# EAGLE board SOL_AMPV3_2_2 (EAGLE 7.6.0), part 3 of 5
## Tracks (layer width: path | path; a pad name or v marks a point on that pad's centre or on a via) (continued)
D13:N$7  (via drill 0.4) (continued)
  BOTTOM 0.254: D13:C35.2 44.85,129.65 44.83,129.67 44.83,129.91 | 44.83,129.91 D13:R39.1 | 44.83,129.91 47.55,129.91 v47.69,130.05
D13:N$10
  Top 0.406: D13:R41.1 30.97,127.93 D13:C41.1
D13:R31
  Top 0.406: D13:R31.1 30.97,135.03 D13:C31.1
D13:VB+
  Top 0.406: D13:R37.2 27.05,133.22 27.37,132.91 27.37,132.59 | 27.37,132.59 27.37,131.97 D13:R36.1 | D13:C36.1 27.37,132.59
D13:VB-  (via drill 0.4)
  Top 0.406: D13:C46.1 28.74,130.68 D13:R46.2 27.37,130.67 27.37,129.73 27.05,129.41 D13:R47.1 26.84,129.09 v25.46,129.41
  BOTTOM 0.406: D13:R50.2 25.48,129.43 v25.46,129.41
D13:VCOM  (via drill 0.4)
  Top 0.254: D13:U1.2 41.33,130.03 41.34,130.05 41.34,130.37 41.02,130.68 v39.43,131
  BOTTOM 0.254: v39.43,131 D13:C7.1 38.19,129.11 D13:R1.2
D14:AMP+
  Top 0.254: 89.58,113.84 86.42,113.86 86.12,114.16 D14:C43.2 85.38,114.16 D14:R43.2 | 89.58,113.84 89.6,114.49 89.6,115.3 D14:U1.4 | 89.58,113.84 89.6,113.86 D14:C44.1 D14:R44.1 D14:R61.2
D14:AMP-
  Top 0.254: D14:R33.2 85.35,120.22 D14:C33.2 86.44,120.22 87.06,120.84 89.61,120.84 | 89.61,120.84 D14:U1.5 | 89.61,120.84 91.49,120.84 D14:R34.1 D14:C34.1 D14:R51.2
D14:FB+
  Top 0.254: D14:R32.1 D14:R33.1 81.66,120.84 D14:C32.2 D14:R31.2
D14:FB-
  Top 0.254: D14:R43.1 83.03,115.44 | 83.03,115.44 D14:R42.1 | D14:R41.2 D14:C42.2 81.66,115.44 83.03,115.44
D14:N$1  (via drill 0.4)
  Top 0.254: D14:R51.1 93.61,117.98 | 93.61,117.98 D14:R45.1 | v94.36,117.98 93.61,117.98
  BOTTOM 0.254: v94.36,117.98 94.09,118.25 D14:R49.1 93.11,118.27 D14:C45.2
D14:N$4
  Top 0.254: D14:U1.1 85.96,115.32 D14:C43.1 85.77,115.14 84.84,116.08 D14:R42.2
D14:N$5
  Top 0.254: D14:U1.8 87.5,119.38 87.38,119.25 87.06,119.25 86.74,118.94 86.12,118.94 D14:C33.1 85.04,118.92 D14:R32.2
D14:N$7  (via drill 0.4)
  Top 0.254: D14:R61.1 v94.68,116.08 95.31,116.71 95.31,118.62 D14:R35.2
  BOTTOM 0.254: v94.68,116.08 93.41,114.81 D14:C35.2 91.82,114.82 91.82,116.08 91.58,116.32 D14:R39.1
D14:N$10
  Top 0.406: D14:R41.1 77.96,113.96 D14:C41.1
D14:R31
  Top 0.406: D14:R31.1 77.96,121.06 D14:C31.1
D14:VB+
  Top 0.406: D14:R37.2 74.04,119.25 74.36,118.94 74.36,118.62 | 74.36,118.62 74.36,118 D14:R36.1 | D14:C36.1 74.36,118.62
D14:VB-  (via drill 0.4)
  Top 0.406: D14:C46.1 75.73,116.71 D14:R46.2 74.36,116.7 74.36,115.76 74.04,115.44 D14:R47.1 73.83,115.13 v72.45,115.44
  BOTTOM 0.406: D14:R50.2 72.47,115.46 v72.45,115.44
D14:VCOM  (via drill 0.4)
  Top 0.254: D14:U1.2 88.32,116.06 88.33,116.08 88.33,116.39 88.01,116.71 v86.42,117.03
  BOTTOM 0.254: v86.42,117.03 D14:C7.1 85.18,115.14 D14:R1.2
D15:AMP+
  Top 0.254: 42.59,115.11 39.43,115.13 39.13,115.43 D15:C43.2 38.39,115.43 D15:R43.2 | 42.59,115.11 42.61,115.76 42.61,116.57 D15:U1.4 | 42.59,115.11 42.61,115.13 D15:C44.1 D15:R44.1 D15:R61.2
D15:AMP-
  Top 0.254: D15:R33.2 38.36,121.49 D15:C33.2 39.45,121.49 40.07,122.11 42.62,122.11 | 42.62,122.11 D15:U1.5 | 42.62,122.11 44.5,122.11 D15:R34.1 D15:C34.1 D15:R51.2
D15:FB+
  Top 0.254: D15:R32.1 D15:R33.1 34.67,122.11 D15:C32.2 D15:R31.2
D15:FB-
  Top 0.254: D15:R43.1 36.04,116.71 | 36.04,116.71 D15:R42.1 | D15:R41.2 D15:C42.2 34.67,116.71 36.04,116.71
D15:N$1  (via drill 0.4)
  Top 0.254: D15:R51.1 46.62,119.25 | 46.62,119.25 D15:R45.1 | v47.37,119.25 46.62,119.25
  BOTTOM 0.254: D15:C45.2 46.1,121.14 D15:R49.1 47.1,119.52 v47.37,119.25
D15:N$4
  Top 0.254: D15:U1.1 38.97,116.59 D15:C43.1 38.78,116.41 37.85,117.35 D15:R42.2
D15:N$5
  Top 0.254: D15:U1.8 40.51,120.65 40.39,120.52 40.07,120.52 39.75,120.21 39.13,120.21 D15:C33.1 38.05,120.19 D15:R32.2
D15:N$7  (via drill 0.4)
  Top 0.254: D15:R61.1 v47.69,117.35 48.32,117.98 48.32,119.89 D15:R35.2
  BOTTOM 0.254: D15:R39.1 44.59,117.71 44.96,117.35 44.96,116.19 D15:C35.2 46.42,116.08 v47.69,117.35
D15:N$10
  Top 0.406: D15:R41.1 30.97,115.23 D15:C41.1
D15:R31
  Top 0.406: D15:R31.1 30.97,122.33 D15:C31.1
D15:VB+
  Top 0.406: D15:R37.2 27.05,120.52 27.37,120.21 27.37,119.89 | 27.37,119.89 27.37,119.27 D15:R36.1 | D15:C36.1 27.37,119.89
D15:VB-  (via drill 0.4)
  Top 0.406: D15:C46.1 28.74,117.98 D15:R46.2 27.37,117.97 27.37,117.03 27.05,116.71 D15:R47.1 26.84,116.39 v25.46,116.71
  BOTTOM 0.406: D15:R50.2 25.48,116.73 v25.46,116.71
D15:VCOM  (via drill 0.4)
  Top 0.254: D15:U1.2 41.33,117.33 41.34,117.35 41.34,117.67 41.02,117.98 v39.43,118.3
  BOTTOM 0.254: v39.43,118.3 D15:C7.1 38.19,116.41 D15:R1.2
D16:AMP+
  Top 0.254: 42.59,98.6 39.43,98.61 39.13,98.92 D16:C43.2 38.39,98.92 D16:R43.2 | 42.59,98.6 42.61,99.25 42.61,100.06 D16:U1.4 | 42.59,98.6 42.61,98.61 D16:C44.1 D16:R44.1 D16:R61.2
D16:AMP-
  Top 0.254: D16:R33.2 38.36,104.98 D16:C33.2 39.45,104.98 40.07,105.6 42.62,105.6 | 42.62,105.6 D16:U1.5 | 42.62,105.6 44.5,105.6 D16:R34.1 D16:C34.1 D16:R51.2
D16:FB+
  Top 0.254: D16:R32.1 D16:R33.1 34.67,105.6 D16:C32.2 D16:R31.2
D16:FB-
  Top 0.254: D16:R43.1 36.04,100.2 | 36.04,100.2 D16:R42.1 | D16:R41.2 D16:C42.2 34.67,100.2 36.04,100.2
D16:N$1  (via drill 0.4)
  Top 0.254: D16:R51.1 46.62,102.74 | 46.62,102.74 D16:R45.1 | v47.37,102.74 46.62,102.74
  BOTTOM 0.254: v47.37,102.74 47.1,103.01 D16:R49.1 46.12,103.03 D16:C45.2
D16:N$4
  Top 0.254: D16:U1.1 38.97,100.08 D16:C43.1 38.78,99.9 37.85,100.84 D16:R42.2
D16:N$5
  Top 0.254: D16:U1.8 40.51,104.14 40.39,104.01 40.07,104.01 39.75,103.69 39.13,103.69 D16:C33.1 38.05,103.68 D16:R32.2
D16:N$7  (via drill 0.4)
  Top 0.254: D16:R61.1 v47.69,100.84 48.32,101.47 48.32,103.38 D16:R35.2
  BOTTOM 0.254: D16:R39.1 44.59,101.08 44.83,100.84 | 44.83,100.84 44.83,99.58 D16:C35.2 | 44.83,100.84 v47.69,100.84
D16:N$10
  Top 0.406: D16:R41.1 30.97,98.72 D16:C41.1
D16:R31
  Top 0.406: D16:R31.1 30.97,105.82 D16:C31.1
D16:VB+
  Top 0.406: D16:R37.2 27.05,104.01 27.37,103.69 27.37,103.38 | 27.37,103.38 27.37,102.76 D16:R36.1 | D16:C36.1 27.37,103.38
D16:VB-  (via drill 0.4)
  Top 0.406: D16:C46.1 28.74,101.47 D16:R46.2 27.37,101.46 27.37,100.52 27.05,100.2 D16:R47.1 26.84,99.89 v25.46,100.2
  BOTTOM 0.406: D16:R50.2 25.48,100.22 v25.46,100.2
D16:VCOM  (via drill 0.4)
  Top 0.254: D16:U1.2 41.33,100.83 41.34,100.84 41.34,101.16 41.02,101.47 v39.43,101.79
  BOTTOM 0.254: v39.43,101.79 D16:C7.1 38.19,99.9 D16:R1.2
D17:AMP+
  Top 0.254: 78.79,95.68 75.63,95.69 75.33,96 D17:C43.2 74.59,96 D17:R43.2 | 78.79,95.68 78.8,96.33 78.8,97.14 D17:U1.4 | 78.79,95.68 78.8,95.69 D17:C44.1 D17:R44.1 D17:R61.2
D17:AMP-
  Top 0.254: D17:R33.2 74.56,102.06 D17:C33.2 75.64,102.06 76.26,102.68 78.82,102.68 | 78.82,102.68 D17:U1.5 | 78.82,102.68 80.69,102.68 D17:R34.1 D17:C34.1 D17:R51.2
D17:FB+
  Top 0.254: D17:R32.1 D17:R33.1 70.87,102.68 D17:C32.2 D17:R31.2
D17:FB-
  Top 0.254: D17:R43.1 72.24,97.28 | 72.24,97.28 D17:R42.1 | D17:R41.2 D17:C42.2 70.87,97.28 72.24,97.28
D17:N$1  (via drill 0.4)
  Top 0.254: D17:R51.1 82.82,99.82 | 82.82,99.82 D17:R45.1 | v83.57,99.82 82.82,99.82
  BOTTOM 0.254: v83.57,99.82 83.3,100.09 D17:R49.1 82.31,100.11 D17:C45.2
D17:N$4
  Top 0.254: D17:U1.1 75.17,97.16 D17:C43.1 74.98,96.98 74.04,97.92 D17:R42.2
D17:N$5
  Top 0.254: D17:U1.8 76.71,101.22 76.58,101.09 76.26,101.09 75.95,100.78 75.33,100.78 D17:C33.1 74.24,100.76 D17:R32.2
D17:N$7  (via drill 0.4)
  Top 0.254: D17:R61.1 v83.88,97.92 84.52,98.55 84.52,100.46 D17:R35.2
  BOTTOM 0.305: D17:C35.2 81.03,97.66 81.03,97.92 | D17:R39.1 81.03,97.92 | 81.03,97.92 v83.88,97.92
D17:N$10
  Top 0.406: D17:R41.1 67.17,95.8 D17:C41.1
D17:R31
  Top 0.406: D17:R31.1 67.17,102.89 D17:C31.1
D17:VB+
  Top 0.406: D17:R37.2 63.25,101.09 63.56,100.78 63.56,100.46 | 63.56,100.46 63.56,99.84 D17:R36.1 | D17:C36.1 63.56,100.46
D17:VB-  (via drill 0.4)
  Top 0.406: D17:C46.1 64.94,98.55 D17:R46.2 63.56,98.54 63.56,97.6 63.25,97.28 D17:R47.1 63.03,96.97 v61.66,97.28
  BOTTOM 0.406: D17:R50.2 61.67,97.3 v61.66,97.28
D17:VCOM  (via drill 0.4)
  Top 0.254: D17:U1.2 77.52,97.9 77.53,97.92 77.53,98.23 77.22,98.55 v75.63,98.87
  BOTTOM 0.254: v75.63,98.87 D17:C7.1 74.39,96.98 D17:R1.2
D18:AMP+
  Top 0.254: 42.59,87.42 39.43,87.44 39.13,87.74 D18:C43.2 38.39,87.74 D18:R43.2 | 42.59,87.42 42.61,88.08 42.61,88.89 D18:U1.4 | 42.59,87.42 42.61,87.44 D18:C44.1 D18:R44.1 D18:R61.2
D18:AMP-
  Top 0.254: D18:R33.2 38.36,93.81 D18:C33.2 39.45,93.81 40.07,94.42 42.62,94.42 | 42.62,94.42 D18:U1.5 | 42.62,94.42 44.5,94.42 D18:R34.1 D18:C34.1 D18:R51.2
D18:FB+
  Top 0.254: D18:R32.1 D18:R33.1 34.67,94.42 D18:C32.2 D18:R31.2
D18:FB-
  Top 0.254: D18:R43.1 36.04,89.03 | 36.04,89.03 D18:R42.1 | D18:R41.2 D18:C42.2 34.67,89.03 36.04,89.03
D18:N$1  (via drill 0.4)
  Top 0.254: D18:R51.1 46.62,91.57 | 46.62,91.57 D18:R45.1 | v47.37,91.57 46.62,91.57
  BOTTOM 0.254: D18:C45.2 46.12,91.85 D18:R49.1
  BOTTOM 0.305: D18:R49.1 v47.37,91.57
D18:N$4
  Top 0.254: D18:U1.1 38.97,88.9 D18:C43.1 38.78,88.72 37.85,89.66 D18:R42.2
D18:N$5
  Top 0.254: D18:U1.8 40.51,92.96 40.39,92.84 40.07,92.84 39.75,92.52 39.13,92.52 D18:C33.1 38.05,92.5 D18:R32.2
D18:N$7  (via drill 0.4)
  Top 0.254: D18:R61.1 v47.69,89.66 48.32,90.3 48.32,92.2 D18:R35.2
  BOTTOM 0.254: D18:R39.1 44.96,89.41 | 44.96,89.41 44.96,88.5 D18:C35.2 | 44.96,89.41 47.43,89.41 v47.69,89.66
D18:N$10
  Top 0.406: D18:R41.1 30.97,87.54 D18:C41.1
D18:R31
  Top 0.406: D18:R31.1 30.97,94.64 D18:C31.1
D18:VB+
  Top 0.406: D18:R37.2 27.05,92.84 27.37,92.52 27.37,92.2 | 27.37,92.2 27.37,91.58 D18:R36.1 | D18:C36.1 27.37,92.2
D18:VB-  (via drill 0.4)
  Top 0.406: D18:C46.1 28.74,90.3 D18:R46.2 27.37,90.28 27.37,89.34 27.05,89.03 D18:R47.1 26.84,88.71 v25.46,89.03
  BOTTOM 0.406: D18:R50.2 25.48,89.04 v25.46,89.03
D18:VCOM  (via drill 0.4)
  Top 0.254: D18:U1.2 41.33,89.65 41.34,89.66 41.34,89.98 41.02,90.3 v39.43,90.61
  BOTTOM 0.254: v39.43,90.61 D18:C7.1 38.19,88.72 D18:R1.2
D19:AMP+
  Top 0.254: 78.79,84.25 75.63,84.26 75.33,84.57 D19:C43.2 74.59,84.57 D19:R43.2 | 78.79,84.25 78.8,84.9 78.8,85.71 D19:U1.4 | 78.79,84.25 78.8,84.26 D19:C44.1 D19:R44.1 D19:R61.2
D19:AMP-
  Top 0.254: D19:R33.2 74.56,90.63 D19:C33.2 75.64,90.63 76.26,91.25 78.82,91.25 | 78.82,91.25 D19:U1.5 | 78.82,91.25 80.69,91.25 D19:R34.1 D19:C34.1 D19:R51.2
D19:FB+
  Top 0.254: D19:R32.1 D19:R33.1 70.87,91.25 D19:C32.2 D19:R31.2
D19:FB-
  Top 0.254: D19:R43.1 72.24,85.85 | 72.24,85.85 D19:R42.1 | D19:R41.2 D19:C42.2 70.87,85.85 72.24,85.85
D19:N$1  (via drill 0.4)
  Top 0.254: D19:R51.1 82.82,88.39 | 82.82,88.39 D19:R45.1 | v83.57,88.39 82.82,88.39
  BOTTOM 0.254: v83.57,88.39 83.3,88.66 D19:R49.1 82.31,88.68 D19:C45.2
D19:N$4
  Top 0.254: D19:U1.1 75.17,85.72 D19:C43.1 74.98,85.55 74.04,86.49 D19:R42.2
D19:N$5
  Top 0.254: D19:U1.8 76.71,89.79 76.58,89.66 76.26,89.66 75.95,89.34 75.33,89.34 D19:C33.1 74.24,89.33 D19:R32.2
D19:N$7  (via drill 0.4)
  Top 0.254: D19:R61.1 v83.88,86.49 84.52,87.12 84.52,89.03 D19:R35.2
  BOTTOM 0.254: D19:C35.2 80.9,85.47 80.9,86.47 D19:R39.1 81.39,86.73 81.41,86.74 81.66,86.49 v83.88,86.49
D19:N$10
  Top 0.406: D19:R41.1 67.17,84.37 D19:C41.1
D19:R31
  Top 0.406: D19:R31.1 67.17,91.47 D19:C31.1
D19:VB+
  Top 0.406: D19:R37.2 63.25,89.66 63.56,89.34 63.56,89.03 | 63.56,89.03 63.56,88.41 D19:R36.1 | D19:C36.1 63.56,89.03
D19:VB-  (via drill 0.4)
  Top 0.406: D19:C46.1 64.94,87.12 D19:R46.2 63.56,87.11 63.56,86.17 63.25,85.85 D19:R47.1 63.03,85.53 v61.66,85.85
  BOTTOM 0.406: D19:R50.2 61.67,85.87 v61.66,85.85
D19:VCOM  (via drill 0.4)
  Top 0.254: D19:U1.2 77.52,86.47 77.53,86.49 77.53,86.81 77.22,87.12 v75.63,87.44
  BOTTOM 0.254: v75.63,87.44 D19:C7.1 74.39,85.55 D19:R1.2
D20:AMP+
  Top 0.254: 43.86,71.93 40.7,71.94 40.4,72.25 D20:C43.2 39.66,72.25 D20:R43.2 | 43.86,71.93 43.88,72.58 43.88,73.39 D20:U1.4 | 43.86,71.93 43.88,71.94 D20:C44.1 D20:R44.1 D20:R61.2
D20:AMP-
  Top 0.254: D20:R33.2 39.63,78.31 D20:C33.2 40.72,78.31 41.34,78.93 43.89,78.93 | 43.89,78.93 D20:U1.5 | 43.89,78.93 45.77,78.93 D20:R34.1 D20:C34.1 D20:R51.2
D20:FB+
  Top 0.254: D20:R32.1 D20:R33.1 35.94,78.93 D20:C32.2 D20:R31.2
D20:FB-
  Top 0.254: D20:R43.1 37.31,73.53 | 37.31,73.53 D20:R42.1 | D20:R41.2 D20:C42.2 35.94,73.53 37.31,73.53
D20:N$1  (via drill 0.4)
  Top 0.254: D20:R51.1 47.89,76.07 | 47.89,76.07 D20:R45.1 | v48.64,76.07 47.89,76.07
  BOTTOM 0.254: v48.64,76.07 48.37,76.34 D20:R49.1 47.39,76.36 D20:C45.2
D20:N$4
  Top 0.254: D20:U1.1 40.24,73.41 D20:C43.1 40.05,73.23 39.12,74.17 D20:R42.2
D20:N$5
  Top 0.254: D20:U1.8 41.78,77.47 41.66,77.34 41.34,77.34 41.02,77.03 40.4,77.03 D20:C33.1 39.32,77.01 D20:R32.2
D20:N$7  (via drill 0.4)
  Top 0.254: D20:R61.1 v48.96,74.17 49.59,74.8 49.59,76.71 D20:R35.2
  BOTTOM 0.254: 45.97,74.17 45.97,73.04 D20:C35.2 | D20:R39.1 45.73,74.41 45.97,74.17 | 45.97,74.17 v48.96,74.17
D20:N$10
  Top 0.406: D20:R41.1 32.24,72.05 D20:C41.1
D20:R31
  Top 0.406: D20:R31.1 32.24,79.14 D20:C31.1
D20:VB+
  Top 0.406: D20:R37.2 28.32,77.34 28.64,77.03 28.64,76.71 | 28.64,76.71 28.64,76.09 D20:R36.1 | D20:C36.1 28.64,76.71
D20:VB-  (via drill 0.4)
  Top 0.406: D20:C46.1 30.01,74.8 D20:R46.2 28.64,74.79 28.64,73.85 28.32,73.53 D20:R47.1 28.11,73.22 v26.73,73.53
  BOTTOM 0.406: D20:R50.2 26.75,73.55 v26.73,73.53
D20:VCOM  (via drill 0.4)
  Top 0.254: D20:U1.2 42.6,74.16 42.61,74.17 42.61,74.49 42.29,74.8 v40.7,75.12
  BOTTOM 0.254: v40.7,75.12 D20:C7.1 39.46,73.23 D20:R1.2
D21:AMP+
  Top 0.254: 85.77,69.39 82.61,69.41 82.31,69.71 D21:C43.2 81.57,69.71 D21:R43.2 | 85.77,69.39 85.79,70.04 85.79,70.85 D21:U1.4 | 85.77,69.39 85.79,69.41 D21:C44.1 D21:R44.1 D21:R61.2
D21:AMP-
  Top 0.254: D21:R33.2 81.54,75.77 D21:C33.2 82.63,75.77 83.25,76.39 85.8,76.39 | 85.8,76.39 D21:U1.5 | 85.8,76.39 87.68,76.39 D21:R34.1 D21:C34.1 D21:R51.2
D21:FB+
  Top 0.254: D21:R32.1 D21:R33.1 77.85,76.39 D21:C32.2 D21:R31.2
D21:FB-
  Top 0.254: D21:R43.1 79.22,70.99 | 79.22,70.99 D21:R42.1 | D21:R41.2 D21:C42.2 77.85,70.99 79.22,70.99
D21:N$1  (via drill 0.4)
  Top 0.254: D21:R51.1 89.8,73.53 | 89.8,73.53 D21:R45.1 | v90.55,73.53 89.8,73.53
  BOTTOM 0.254: v90.55,73.53 90.28,73.8 D21:R49.1 89.3,73.83 D21:C45.2
D21:N$4
  Top 0.254: D21:U1.1 82.15,70.87 D21:C43.1 81.96,70.69 81.03,71.63 D21:R42.2
D21:N$5
  Top 0.254: D21:U1.8 83.69,74.93 83.57,74.8 83.25,74.8 82.93,74.49 82.31,74.49 D21:C33.1 81.23,74.47 D21:R32.2
D21:N$7  (via drill 0.4)
  Top 0.254: D21:R61.1 v90.87,71.63 91.5,72.26 91.5,74.17 D21:R35.2
  BOTTOM 0.254: D21:C35.2 87.88,70.5 87.88,71.63 87.63,71.63 D21:R39.1 87.87,71.63 v90.87,71.63
D21:N$10
  Top 0.406: D21:R41.1 74.15,69.51 D21:C41.1
D21:R31
  Top 0.406: D21:R31.1 74.15,76.61 D21:C31.1
D21:VB+
  Top 0.406: D21:R37.2 70.23,74.8 70.55,74.49 70.55,74.17 | 70.55,74.17 70.55,73.55 D21:R36.1 | D21:C36.1 70.55,74.17
D21:VB-  (via drill 0.4)
  Top 0.406: D21:C46.1 71.92,72.26 D21:R46.2 70.55,72.25 70.55,71.31 70.23,70.99 D21:R47.1 70.02,70.67 v68.64,70.99
  BOTTOM 0.406: D21:R50.2 68.66,71.01 v68.64,70.99
D21:VCOM  (via drill 0.4)
  Top 0.254: D21:U1.2 84.51,71.61 84.52,71.63 84.52,71.94 84.2,72.26 v82.61,72.58
  BOTTOM 0.254: v82.61,72.58 D21:C7.1 81.37,70.69 D21:R1.2
D22:AMP+
  Top 0.254: 42.59,60.5 39.43,60.52 39.13,60.82 D22:C43.2 38.39,60.82 D22:R43.2 | 42.59,60.5 42.61,61.15 42.61,61.96 D22:U1.4 | 42.59,60.5 42.61,60.52 D22:C44.1 D22:R44.1 D22:R61.2
D22:AMP-
  Top 0.254: D22:R33.2 38.36,66.88 D22:C33.2 39.45,66.88 40.07,67.5 42.62,67.5 | 42.62,67.5 D22:U1.5 | 42.62,67.5 44.5,67.5 D22:R34.1 D22:C34.1 D22:R51.2
D22:FB+
  Top 0.254: D22:R32.1 D22:R33.1 34.67,67.5 D22:C32.2 D22:R31.2
D22:FB-
  Top 0.254: D22:R43.1 36.04,62.1 | 36.04,62.1 D22:R42.1 | D22:R41.2 D22:C42.2 34.67,62.1 36.04,62.1
D22:N$1  (via drill 0.4)
  Top 0.254: D22:R51.1 46.62,64.64 | 46.62,64.64 D22:R45.1 | v47.37,64.64 46.62,64.64
  BOTTOM 0.254: D22:C45.2 46.1,66.53 D22:R49.1 47.1,64.91 v47.37,64.64
D22:N$4
  Top 0.254: D22:U1.1 38.97,61.98 D22:C43.1 38.78,61.8 37.85,62.74 D22:R42.2
D22:N$5
  Top 0.254: D22:U1.8 40.51,66.04 40.39,65.91 40.07,65.91 39.75,65.6 39.13,65.6 D22:C33.1 38.05,65.58 D22:R32.2
D22:N$7  (via drill 0.4)
  Top 0.254: D22:R61.1 v47.69,62.74 48.32,63.37 48.32,65.28 D22:R35.2
  BOTTOM 0.254: D22:R39.1 44.45,62.99 44.83,62.61 | 44.83,62.61 44.83,61.48 D22:C35.2 | 44.83,62.61 45.99,62.61 D22:R61.1 v47.69,62.74
D22:N$10
  Top 0.406: D22:R41.1 30.97,60.62 D22:C41.1
D22:R31
  Top 0.406: D22:R31.1 30.97,67.72 D22:C31.1
D22:VB+
  Top 0.406: D22:R37.2 27.05,65.91 27.37,65.6 27.37,65.28 | 27.37,65.28 27.37,64.66 D22:R36.1 | D22:C36.1 27.37,65.28
D22:VB-  (via drill 0.4)
  Top 0.406: D22:C46.1 28.74,63.37 D22:R46.2 27.37,63.36 27.37,62.42 27.05,62.1 D22:R47.1 26.84,61.78 v25.46,62.1
  BOTTOM 0.406: D22:R50.2 25.48,62.12 v25.46,62.1
D22:VCOM  (via drill 0.4)
  Top 0.254: D22:U1.2 41.33,62.73 41.34,62.74 41.34,63.06 41.02,63.37 v39.43,63.69
  BOTTOM 0.254: v39.43,63.69 D22:C7.1 38.19,61.8 D22:R1.2
D23:AMP+
  Top 0.254: 89.58,57.96 86.42,57.98 86.12,58.28 D23:C43.2 85.38,58.28 D23:R43.2 | 89.58,57.96 89.6,58.61 89.6,59.42 D23:U1.4 | 89.58,57.96 89.6,57.98 D23:C44.1 D23:R44.1 D23:R61.2
D23:AMP-
  Top 0.254: D23:R33.2 85.35,64.34 D23:C33.2 86.44,64.34 87.06,64.96 89.61,64.96 | 89.61,64.96 D23:U1.5 | 89.61,64.96 91.49,64.96 D23:R34.1 D23:C34.1 D23:R51.2
D23:FB+
  Top 0.254: D23:R32.1 D23:R33.1 81.66,64.96 D23:C32.2 D23:R31.2
D23:FB-
  Top 0.254: D23:R43.1 83.03,59.56 | 83.03,59.56 D23:R42.1 | D23:R41.2 D23:C42.2 81.66,59.56 83.03,59.56
D23:N$1  (via drill 0.4)
  Top 0.254: D23:R51.1 93.61,62.1 | 93.61,62.1 D23:R45.1 | v94.36,62.1 93.61,62.1
  BOTTOM 0.305: D23:C45.2 93.09,63.99 D23:R49.1 93.46,62.37 94.23,62.23 v94.36,62.1
D23:N$4
  Top 0.254: D23:U1.1 85.96,59.44 D23:C43.1 85.77,59.26 84.84,60.2 D23:R42.2
D23:N$5
  Top 0.254: D23:U1.8 87.5,63.5 87.38,63.37 87.06,63.37 86.74,63.06 86.12,63.06 D23:C33.1 85.04,63.04 D23:R32.2
D23:N$7  (via drill 0.4)
  Top 0.254: D23:R61.1 v94.68,60.2 95.31,60.83 95.31,62.74 D23:R35.2
  BOTTOM 0.305: D23:R39.1 91.69,60.2 | 91.69,60.2 91.69,59.07 D23:C35.2 | 91.69,60.2 v94.68,60.2
D23:N$10
  Top 0.406: D23:R41.1 77.96,58.08 D23:C41.1
D23:R31
  Top 0.406: D23:R31.1 77.96,65.17 D23:C31.1
D23:VB+
  Top 0.406: D23:R37.2 74.04,63.37 74.36,63.06 74.36,62.74 | 74.36,62.74 74.36,62.12 D23:R36.1 | D23:C36.1 74.36,62.74
D23:VB-  (via drill 0.4)
  Top 0.406: D23:C46.1 75.73,60.83 D23:R46.2 74.36,60.82 74.36,59.88 74.04,59.56 D23:R47.1 73.83,59.24 v72.45,59.56
  BOTTOM 0.406: D23:R50.2 72.47,59.58 v72.45,59.56
D23:VCOM  (via drill 0.4)
  Top 0.254: D23:U1.2 88.32,60.19 88.33,60.2 88.33,60.52 88.01,60.83 v86.42,61.15
  BOTTOM 0.254: v86.42,61.15 D23:C7.1 85.18,59.26 D23:R1.2
D24:AMP+
  Top 0.254: 42.59,45.26 39.43,45.28 39.13,45.58 D24:C43.2 38.39,45.58 D24:R43.2 | 42.59,45.26 42.61,45.91 42.61,46.72 D24:U1.4 | 42.59,45.26 42.61,45.28 D24:C44.1 D24:R44.1 D24:R61.2
D24:AMP-
  Top 0.254: D24:R33.2 38.36,51.64 D24:C33.2 39.45,51.64 40.07,52.26 42.62,52.26 | 42.62,52.26 D24:U1.5 | 42.62,52.26 44.5,52.26 D24:R34.1 D24:C34.1 D24:R51.2
D24:FB+
  Top 0.254: D24:R32.1 D24:R33.1 34.67,52.26 D24:C32.2 D24:R31.2
D24:FB-
  Top 0.254: D24:R43.1 36.04,46.86 | 36.04,46.86 D24:R42.1 | D24:R41.2 D24:C42.2 34.67,46.86 36.04,46.86
D24:N$1  (via drill 0.4)
  Top 0.254: D24:R51.1 46.62,49.4 | 46.62,49.4 D24:R45.1 | v47.37,49.4 46.62,49.4
  BOTTOM 0.254: v47.37,49.4 47.1,49.67 D24:R49.1 46.12,49.69 D24:C45.2
D24:N$4
  Top 0.254: D24:U1.1 38.97,46.74 D24:C43.1 38.78,46.56 37.85,47.5 D24:R42.2
D24:N$5
  Top 0.254: D24:U1.8 40.51,50.8 40.39,50.67 40.07,50.67 39.75,50.35 39.13,50.35 D24:C33.1 38.05,50.34 D24:R32.2
D24:N$7  (via drill 0.4)
  Top 0.254: D24:R61.1 v47.69,47.5 48.32,48.13 48.32,50.04 D24:R35.2
  BOTTOM 0.254: 44.7,47.5 44.7,46.37 D24:C35.2 | D24:R39.1 44.7,47.5 | 44.7,47.5 v47.69,47.5
D24:N$10
  Top 0.406: D24:R41.1 30.97,45.38 D24:C41.1
D24:R31
  Top 0.406: D24:R31.1 30.97,52.48 D24:C31.1
D24:VB+
  Top 0.406: D24:R37.2 27.05,50.67 27.37,50.35 27.37,50.04 | 27.37,50.04 27.37,49.42 D24:R36.1 | D24:C36.1 27.37,50.04
D24:VB-  (via drill 0.4)
  Top 0.406: D24:C46.1 28.74,48.13 D24:R46.2 27.37,48.12 27.37,47.18 27.05,46.86 D24:R47.1 26.84,46.55 v25.46,46.86
  BOTTOM 0.406: D24:R50.2 25.48,46.88 v25.46,46.86
D24:VCOM  (via drill 0.4)
  Top 0.254: D24:U1.2 41.33,47.48 41.34,47.5 41.34,47.82 41.02,48.13 v39.43,48.45
  BOTTOM 0.254: v39.43,48.45 D24:C7.1 38.19,46.56 D24:R1.2
D25:AMP+
  Top 0.254: 89.58,43.23 86.42,43.24 86.12,43.55 D25:C43.2 85.38,43.55 D25:R43.2 | 89.58,43.23 89.6,43.88 89.6,44.69 D25:U1.4 | 89.58,43.23 89.6,43.24 D25:C44.1 D25:R44.1 D25:R61.2
D25:AMP-
  Top 0.254: D25:R33.2 85.35,49.61 D25:C33.2 86.44,49.61 87.06,50.23 89.61,50.23 | 89.61,50.23 D25:U1.5 | 89.61,50.23 91.49,50.23 D25:R34.1 D25:C34.1 D25:R51.2
D25:FB+
  Top 0.254: D25:R32.1 D25:R33.1 81.66,50.23 D25:C32.2 D25:R31.2
D25:FB-
  Top 0.254: D25:R43.1 83.03,44.83 | 83.03,44.83 D25:R42.1 | D25:R41.2 D25:C42.2 81.66,44.83 83.03,44.83
D25:N$1  (via drill 0.4)
  Top 0.254: D25:R51.1 93.11,47.37 | 93.11,47.37 D25:R45.1 | v94.36,47.37 93.11,47.37
  BOTTOM 0.254: v94.36,47.37 94.09,47.64 D25:R49.1 93.11,47.66 D25:C45.2
D25:N$4
  Top 0.254: D25:U1.1 85.96,44.7 D25:C43.1 85.77,44.53 84.84,45.47 D25:R42.2
D25:N$5
  Top 0.254: D25:U1.8 87.5,48.77 87.38,48.64 87.06,48.64 86.74,48.32 86.12,48.32 D25:C33.1 85.04,48.31 D25:R32.2
D25:N$7  (via drill 0.4)
  Top 0.254: D25:R61.1 v94.68,45.47 95.31,46.1 95.31,48.01 D25:R35.2
  BOTTOM 0.254: 91.69,45.47 91.69,44.34 D25:C35.2 | D25:R39.1 91.69,45.47 | 91.69,45.47 v94.68,45.47
D25:N$10
  Top 0.406: D25:R41.1 77.96,43.35 D25:C41.1
D25:R31
  Top 0.406: D25:R31.1 77.96,50.44 D25:C31.1
D25:VB+
  Top 0.406: D25:R37.2 74.04,48.64 74.36,48.32 74.36,48.01 | 74.36,48.01 74.36,47.39 D25:R36.1 | D25:C36.1 74.36,48.01
D25:VB-  (via drill 0.4)
  Top 0.406: D25:C46.1 75.73,46.1 D25:R46.2 74.36,46.09 74.36,45.15 74.04,44.83 D25:R47.1 73.83,44.51 v72.45,44.83
  BOTTOM 0.406: D25:R50.2 72.47,44.85 v72.45,44.83
D25:VCOM  (via drill 0.4)
  Top 0.254: D25:U1.2 88.32,45.45 88.33,45.47 88.33,45.78 88.01,46.1 v86.42,46.42
  BOTTOM 0.254: v86.42,46.42 D25:C7.1 85.18,44.53 D25:R1.2
D26:AMP+
  Top 0.254: 42.59,33.83 39.43,33.85 39.13,34.15 D26:C43.2 38.39,34.15 D26:R43.2 | 42.59,33.83 42.61,34.48 42.61,35.29 D26:U1.4 | 42.59,33.83 42.61,33.85 D26:C44.1 D26:R44.1 D26:R61.2
D26:AMP-
  Top 0.254: D26:R33.2 38.36,40.21 D26:C33.2 39.45,40.21 40.07,40.83 42.62,40.83 | 42.62,40.83 D26:U1.5 | 42.62,40.83 44.5,40.83 D26:R34.1 D26:C34.1 D26:R51.2
D26:FB+
  Top 0.254: D26:R32.1 D26:R33.1 34.67,40.83 D26:C32.2 D26:R31.2
D26:FB-
  Top 0.254: D26:R43.1 36.04,35.43 | 36.04,35.43 D26:R42.1 | D26:R41.2 D26:C42.2 34.67,35.43 36.04,35.43
D26:N$1  (via drill 0.4)
  Top 0.254: D26:R51.1 46.62,37.97 | 46.62,37.97 D26:R45.1 | v47.37,37.97 46.62,37.97
  BOTTOM 0.254: v47.37,37.97 47.1,38.24 D26:R49.1 46.12,38.26 D26:C45.2
D26:N$4
  Top 0.254: D26:U1.1 38.97,35.31 D26:C43.1 38.78,35.13 37.85,36.07 D26:R42.2
D26:N$5
  Top 0.254: D26:U1.8 40.51,39.37 40.39,39.24 40.07,39.24 39.75,38.92 39.13,38.92 D26:C33.1 38.05,38.91 D26:R32.2
D26:N$7  (via drill 0.4)
  Top 0.254: D26:R61.1 v47.69,36.07 48.32,36.7 48.32,38.61 D26:R35.2
  BOTTOM 0.254: D26:C35.2 44.7,34.94 44.7,36.2 44.59,36.31 D26:R39.1 44.45,36.07 v47.69,36.07
D26:N$10
  Top 0.406: D26:R41.1 30.97,33.95 D26:C41.1
D26:R31
  Top 0.406: D26:R31.1 30.97,41.05 D26:C31.1
D26:VB+
  Top 0.406: D26:R37.2 27.05,39.24 27.37,38.92 27.37,38.61 | 27.37,38.61 27.37,37.99 D26:R36.1 | D26:C36.1 27.37,38.61
D26:VB-  (via drill 0.4)
  Top 0.406: D26:C46.1 28.74,36.7 D26:R46.2 27.37,36.69 27.37,35.75 27.05,35.43 D26:R47.1 26.84,35.12 v25.46,35.43
  BOTTOM 0.406: D26:R50.2 25.48,35.45 v25.46,35.43
D26:VCOM  (via drill 0.4)
  Top 0.254: D26:U1.2 41.33,36.05 41.34,36.07 41.34,36.39 41.02,36.7 v39.43,37.02
  BOTTOM 0.254: v39.43,37.02 D26:C7.1 38.19,35.13 D26:R1.2
D27:AMP+
  Top 0.254: 89.58,31.8 86.42,31.81 86.12,32.12 D27:C43.2 85.38,32.12 D27:R43.2 | 89.58,31.8 89.6,32.45 89.6,33.26 D27:U1.4 | 89.58,31.8 89.6,31.81 D27:C44.1 D27:R44.1 D27:R61.2
D27:AMP-
  Top 0.254: D27:R33.2 85.35,38.18 D27:C33.2 86.44,38.18 87.06,38.8 89.61,38.8 | 89.61,38.8 D27:U1.5 | 89.61,38.8 91.49,38.8 D27:R34.1 D27:C34.1 D27:R51.2
D27:FB+
  Top 0.254: D27:R32.1 D27:R33.1 81.66,38.8 D27:C32.2 D27:R31.2
D27:FB-
  Top 0.254: D27:R43.1 83.03,33.4 | 83.03,33.4 D27:R42.1 | D27:R41.2 D27:C42.2 81.66,33.4 83.03,33.4
D27:N$1  (via drill 0.4)
  Top 0.254: D27:R51.1 93.61,35.94 | 93.61,35.94 D27:R45.1 | v94.36,35.94 93.61,35.94
  BOTTOM 0.254: v94.36,35.94 94.09,36.21 D27:R49.1 93.11,36.23 D27:C45.2
D27:N$4
  Top 0.254: D27:U1.1 85.96,33.27 D27:C43.1 85.77,33.1 84.84,34.04 D27:R42.2
D27:N$5
  Top 0.254: D27:U1.8 87.5,37.34 87.38,37.21 87.06,37.21 86.74,36.89 86.12,36.89 D27:C33.1 85.04,36.88 D27:R32.2
D27:N$7  (via drill 0.4)
  Top 0.254: D27:R61.1 v94.68,34.04 95.31,34.67 95.31,36.58 D27:R35.2
  BOTTOM 0.254: 91.69,34.04 91.69,32.91 D27:C35.2 | D27:R39.1 91.69,34.04 | 91.69,34.04 v94.68,34.04
D27:N$10
  Top 0.406: D27:R41.1 77.96,31.92 D27:C41.1
D27:R31
  Top 0.406: D27:R31.1 77.96,39.01 D27:C31.1
D27:VB+
  Top 0.406: D27:R37.2 74.04,37.21 74.36,36.89 74.36,36.58 | 74.36,36.58 74.36,35.96 D27:R36.1 | D27:C36.1 74.36,36.58
D27:VB-  (via drill 0.4)
  Top 0.406: D27:C46.1 75.73,34.67 D27:R46.2 74.36,34.66 74.36,33.72 74.04,33.4 D27:R47.1 73.83,33.08 v72.45,33.4
  BOTTOM 0.406: D27:R50.2 72.47,33.42 v72.45,33.4
D27:VCOM  (via drill 0.4)
  Top 0.254: D27:U1.2 88.32,34.02 88.33,34.04 88.33,34.35 88.01,34.67 v86.42,34.99
  BOTTOM 0.254: v86.42,34.99 D27:C7.1 85.18,33.1 D27:R1.2
D28:AMP+
  Top 0.254: 43.23,20.5 40.07,20.51 39.77,20.81 D28:C43.2 39.03,20.81 D28:R43.2 | 43.23,20.5 43.24,21.14 43.24,21.96 D28:U1.4 | 43.23,20.5 43.24,20.51 D28:C44.1 D28:R44.1 D28:R61.2
D28:AMP-
  Top 0.254: D28:R33.2 39,26.88 D28:C33.2 40.08,26.88 40.7,27.5 43.26,27.5 | 43.26,27.5 D28:U1.5 | 43.26,27.5 45.13,27.5 D28:R34.1 D28:C34.1 D28:R51.2
D28:FB+
  Top 0.254: D28:R32.1 D28:R33.1 35.31,27.5 D28:C32.2 D28:R31.2
D28:FB-
  Top 0.254: D28:R43.1 36.68,22.1 | 36.68,22.1 D28:R42.1 | D28:R41.2 D28:C42.2 35.31,22.1 36.68,22.1
D28:N$1  (via drill 0.4)
  Top 0.254: D28:R51.1 47.26,24.64 | 47.26,24.64 D28:R45.1 | v48.01,24.64 47.26,24.64
  BOTTOM 0.254: v48.01,24.64 47.74,24.91 D28:R49.1 46.75,24.92 D28:C45.2
D28:N$4
  Top 0.254: D28:U1.1 39.61,21.97 D28:C43.1 39.42,21.8 38.48,22.73 D28:R42.2
D28:N$5
  Top 0.254: D28:U1.8 41.15,26.04 41.02,25.91 40.7,25.91 40.39,25.59 39.77,25.59 D28:C33.1 38.68,25.58 D28:R32.2
D28:N$7  (via drill 0.4)
  Top 0.254: D28:R61.1 v48.32,22.73 48.96,23.37 48.96,25.27 D28:R35.2
  BOTTOM 0.254: D28:R39.1 45.1,22.97 45.34,22.73 | 45.34,22.73 45.34,21.61 D28:C35.2 | 45.34,22.73 v48.32,22.73
D28:N$10
  Top 0.406: D28:R41.1 31.61,20.61 D28:C41.1
D28:R31
  Top 0.406: D28:R31.1 31.61,27.71 D28:C31.1
D28:VB+
  Top 0.406: D28:R37.2 27.69,25.91 28,25.59 28,25.27 | 28,25.27 28,24.65 D28:R36.1 | D28:C36.1 28,25.27
D28:VB-  (via drill 0.4)
  Top 0.406: D28:C46.1 29.38,23.37 D28:R46.2 28,23.35 28,22.42 27.69,22.1 D28:R47.1 27.47,21.78 v26.1,22.1
  BOTTOM 0.406: D28:R50.2 26.11,22.11 v26.1,22.1
D28:VCOM  (via drill 0.4)
  Top 0.254: D28:U1.2 41.96,22.72 41.97,22.73 41.97,23.05 41.66,23.37 v40.07,23.69
  BOTTOM 0.254: v40.07,23.69 D28:C7.1 38.83,21.8 D28:R1.2
D29:AMP+
  Top 0.254: 89.58,17.57 86.42,17.59 86.12,17.89 D29:C43.2 85.38,17.89 D29:R43.2 | 89.58,17.57 89.6,18.22 89.6,19.04 D29:U1.4 | 89.58,17.57 89.6,17.59 D29:C44.1 D29:R44.1 D29:R61.2
D29:AMP-
  Top 0.254: D29:R33.2 85.35,23.95 D29:C33.2 86.44,23.95 87.06,24.57 89.61,24.57 | 89.61,24.57 D29:U1.5 | 89.61,24.57 91.49,24.57 D29:R34.1 D29:C34.1 D29:R51.2
D29:FB+
  Top 0.254: D29:R32.1 D29:R33.1 81.66,24.57 D29:C32.2 D29:R31.2
D29:FB-
  Top 0.254: D29:R43.1 83.03,19.18 | 83.03,19.18 D29:R42.1 | D29:R41.2 D29:C42.2 81.66,19.18 83.03,19.18
D29:N$1  (via drill 0.4)
  Top 0.254: D29:R51.1 93.61,21.72 | 93.61,21.72 D29:R45.1 | v94.36,21.72 93.61,21.72
  BOTTOM 0.254: v94.36,21.72 94.09,21.99 D29:R49.1 93.11,22 D29:C45.2
D29:N$4
  Top 0.254: D29:U1.1 85.96,19.05 D29:C43.1 85.77,18.88 84.84,19.81 D29:R42.2
D29:N$5
  Top 0.254: D29:U1.8 87.5,23.11 87.38,22.99 87.06,22.99 86.74,22.67 86.12,22.67 D29:C33.1 85.04,22.65 D29:R32.2
D29:N$7  (via drill 0.4)
  Top 0.254: D29:R61.1 v94.68,19.81 95.31,20.45 95.31,22.35 D29:R35.2
  BOTTOM 0.254: D29:R39.1 91.69,19.81 | 91.69,19.81 91.69,18.68 D29:C35.2 | 91.69,19.81 v94.68,19.81
D29:N$10
  Top 0.406: D29:R41.1 77.96,17.69 D29:C41.1
D29:R31
  Top 0.406: D29:R31.1 77.96,24.79 D29:C31.1
D29:VB+
  Top 0.406: D29:R37.2 74.04,22.99 74.36,22.67 74.36,22.35 | 74.36,22.35 74.36,21.73 D29:R36.1 | D29:C36.1 74.36,22.35
D29:VB-  (via drill 0.4)
  Top 0.406: D29:C46.1 75.73,20.45 D29:R46.2 74.36,20.43 74.36,19.49 74.04,19.18 D29:R47.1 73.83,18.86 v72.45,19.18
  BOTTOM 0.406: D29:R50.2 72.47,19.19 v72.45,19.18
D29:VCOM  (via drill 0.4)
  Top 0.254: D29:U1.2 88.32,19.8 88.33,19.81 88.33,20.13 88.01,20.45 v86.42,20.77
  BOTTOM 0.254: v86.42,20.77 D29:C7.1 85.18,18.88 D29:R1.2
D30:AMP+
  Top 0.254: 43.23,9.07 40.07,9.08 39.77,9.38 D30:C43.2 39.03,9.38 D30:R43.2 | 43.23,9.07 43.24,9.72 43.24,10.53 D30:U1.4 | 43.23,9.07 43.24,9.08 D30:C44.1 D30:R44.1 D30:R61.2
D30:AMP-
  Top 0.254: D30:R33.2 39,15.45 D30:C33.2 40.08,15.45 40.7,16.07 43.26,16.07 | 43.26,16.07 D30:U1.5 | 43.26,16.07 45.13,16.07 D30:R34.1 D30:C34.1 D30:R51.2
D30:FB+
  Top 0.254: D30:R32.1 D30:R33.1 35.31,16.07 D30:C32.2 D30:R31.2
D30:FB-
  Top 0.254: D30:R43.1 36.68,10.67 | 36.68,10.67 D30:R42.1 | D30:R41.2 D30:C42.2 35.31,10.67 36.68,10.67
D30:N$1  (via drill 0.4)
  Top 0.254: D30:R51.1 47.26,13.21 | 47.26,13.21 D30:R45.1 | v48.01,13.21 47.26,13.21
  BOTTOM 0.254: D30:C45.2 46.75,13.49 | 46.75,13.49 D30:R49.1 | 46.75,13.49 47.72,13.49 v48.01,13.21
D30:N$4
  Top 0.254: D30:U1.1 39.61,10.54 D30:C43.1 39.42,10.37 38.48,11.3 D30:R42.2
D30:N$5
  Top 0.254: D30:U1.8 41.15,14.61 41.02,14.48 40.7,14.48 40.39,14.16 39.77,14.16 D30:C33.1 38.68,14.15 D30:R32.2
D30:N$7  (via drill 0.4)
  Top 0.254: D30:R61.1 v48.32,11.3 48.96,11.94 48.96,13.84 D30:R35.2
  BOTTOM 0.254: 45.48,11.3 D30:C35.2 | 45.48,11.3 v48.32,11.3 | D30:R39.1 45.24,11.54 45.48,11.3
D30:N$10
  Top 0.406: D30:R41.1 31.61,9.18 D30:C41.1
D30:R31
  Top 0.406: D30:R31.1 31.61,16.28 D30:C31.1
D30:VB+
  Top 0.406: D30:R37.2 27.69,14.48 28,14.16 28,13.84 | 28,13.84 28,13.22 D30:R36.1 | D30:C36.1 28,13.84
D30:VB-  (via drill 0.4)
  Top 0.406: D30:C46.1 29.38,11.94 D30:R46.2 28,11.92 28,10.99 27.69,10.67 D30:R47.1 27.47,10.35 v26.1,10.67
  BOTTOM 0.406: D30:R50.2 26.11,10.68 v26.1,10.67
D30:VCOM  (via drill 0.4)
  Top 0.254: D30:U1.2 41.96,11.29 41.97,11.3 41.97,11.62 41.66,11.94 v40.07,12.26
  BOTTOM 0.254: v40.07,12.26 D30:C7.1 38.83,10.37 D30:R1.2
D31:AMP+
  Top 0.254: 89.58,5.89 86.42,5.91 86.12,6.21 D31:C43.2 85.38,6.21 D31:R43.2 | 89.58,5.89 89.6,6.54 89.6,7.35 D31:U1.4 | 89.58,5.89 89.6,5.91 D31:C44.1 D31:R44.1 D31:R61.2
D31:AMP-
  Top 0.254: D31:R33.2 85.35,12.27 D31:C33.2 86.44,12.27 87.06,12.89 89.61,12.89 | 89.61,12.89 D31:U1.5 | 89.61,12.89 91.49,12.89 D31:R34.1 D31:C34.1 D31:R51.2
D31:FB+
  Top 0.254: D31:R32.1 D31:R33.1 81.66,12.89 D31:C32.2 D31:R31.2
D31:FB-
  Top 0.254: D31:R43.1 83.03,7.49 | 83.03,7.49 D31:R42.1 | D31:R41.2 D31:C42.2 81.66,7.49 83.03,7.49
D31:N$1  (via drill 0.4)
  Top 0.254: D31:R51.1 93.61,10.03 | 93.61,10.03 D31:R45.1 | v94.36,10.03 93.61,10.03
  BOTTOM 0.254: v94.36,10.03 94.09,10.3 D31:R49.1 93.11,10.32 D31:C45.2
D31:N$4
  Top 0.254: D31:U1.1 85.96,7.37 D31:C43.1 85.77,7.19 84.84,8.13 D31:R42.2
D31:N$5
  Top 0.254: D31:U1.8 87.5,11.43 87.38,11.3 87.06,11.3 86.74,10.99 86.12,10.99 D31:C33.1 85.04,10.97 D31:R32.2
D31:N$7  (via drill 0.4)
  Top 0.254: D31:R61.1 v94.68,8.13 95.31,8.76 95.31,10.67 D31:R35.2
  BOTTOM 0.254: 91.69,8.13 91.69,7 D31:C35.2 | D31:R39.1 91.69,8.13 | 91.69,8.13 v94.68,8.13
D31:N$10
  Top 0.406: D31:R41.1 77.96,6.01 D31:C41.1
D31:R31
  Top 0.406: D31:R31.1 77.96,13.11 D31:C31.1
D31:VB+
  Top 0.406: D31:R37.2 74.04,11.3 74.36,10.99 74.36,10.67 | 74.36,10.67 74.36,10.05 D31:R36.1 | D31:C36.1 74.36,10.67
D31:VB-  (via drill 0.4)
  Top 0.406: D31:C46.1 75.73,8.76 D31:R46.2 74.36,8.75 74.36,7.81 74.04,7.49 D31:R47.1 73.83,7.18 v72.45,7.49
  BOTTOM 0.406: D31:R50.2 72.47,7.51 v72.45,7.49
D31:VCOM  (via drill 0.4)
  Top 0.254: D31:U1.2 88.32,8.12 88.33,8.13 88.33,8.45 88.01,8.76 v86.42,9.08
  BOTTOM 0.254: v86.42,9.08 D31:C7.1 85.18,7.19 D31:R1.2
GND  (via drill 0.4, 0.5, 0.6)
  Top 0.254: D0:R38.2 49.28,209.04 | 49.28,209.04 v49.28,208.47 49.28,206.9 D0:R48.1 49.01,206.63 | D1:R38.2 v96.27,206.19 96.27,204.61 D1:R48.1 | D2:R38.2 v49.28,197.04 49.28,196.47 49.28,195.47 D2:R48.1 | D3:R38.2 v96.27,194.25 | v96.27,194.25 96.27,192.67 D3:R48.1 | D4:R38.2 v49.28,181.8 | v49.28,181.8 49.28,180.34 49.28,180.23 D4:R48.1 | D5:R38.2 v96.27,179.26 | v96.27,179.26 96.27,177.69 D5:R48.1 | D6:R38.2 v49.28,169.1 49.28,167.53 D6:R48.1 | D7:R38.2 v96.27,167.83 | v96.27,167.83 96.27,166.26 D7:R48.1 | D8:R38.2 v49.28,156.4 49.28,154.83 D8:R48.1 | D9:R38.2 v96.27,155.13 | v96.27,155.13 96.27,153.56 D9:R48.1 | D10:R38.2 v51.82,143.06 | v51.82,143.06 51.82,141.49 D10:R48.1 | D11:R38.2 v96.27,142.43 | v96.27,142.43 96.27,140.86 D11:R48.1 | D13:R38.2 v49.28,131 | v49.28,131 49.28,129.43 D13:R48.1 | D12:R38.2 v96.27,132.27 | v96.27,132.27 96.27,130.7 D12:R48.1 | D15:R38.2 v49.28,118.3 | v49.28,118.3 49.28,116.84 49.28,116.73 D15:R48.1 | D14:R38.2 v96.27,117.03 | v96.27,117.03 96.27,115.46 D14:R48.1 | D16:R38.2 v49.28,101.79 | v49.28,101.79 49.28,100.58 | 49.28,100.58 49.28,100.22 D16:R48.1 | D17:R38.2 v85.47,98.87 | v85.47,98.87 85.47,97.3 D17:R48.1 | D18:R38.2 v49.28,90.61 | v49.28,90.61 49.28,89.04 D18:R48.1 49.18,88.95 | D19:R38.2 v85.47,87.44 85.47,85.87 D19:R48.1 | D20:R38.2 v50.55,75.12 | v50.55,75.12 50.55,74.17 50.55,73.55 D20:R48.1 | D21:R38.2 v92.46,72.58 92.46,71.01 D21:R48.1 | D22:R38.2 v49.28,63.69 | v49.28,63.69 49.28,62.12 D22:R48.1 49.18,62.03 | D23:R38.2 v96.27,61.15 96.27,59.58 D23:R48.1 | D24:R38.2 49.28,49.15 v49.28,48.45 49.28,46.88 D24:R48.1 | D25:R38.2 v96.27,46.42 96.27,44.85 D25:R48.1 | D26:R38.2 v49.28,37.02
  Top 0.254: v49.28,37.02 49.28,35.45 D26:R48.1 | D27:R38.2 v96.27,34.99 96.27,33.42 D27:R48.1 | D28:R38.2 v49.91,23.69 | v49.91,23.69 49.91,22.11 D28:R48.1 | D29:R38.2 v96.27,20.77 96.27,19.19 D29:R48.1 | D30:R38.2 v49.91,12.26 49.91,10.68 D30:R48.1 | D31:R38.2 v96.27,9.08 | v96.27,9.08 96.27,8.13 | 96.27,8.13 96.27,7.51 D31:R48.1 | U5.2 119.38,201.68 v119.63,202.56 | C20.2 v120.27,195.58 | U20.5 U20.4 | U13.2 122.17,78.99 v122.05,78.61 | U3.13 112.53,7.74 112.65,7.62 v113.28,7.62 | U3.14 113.03,7.87 v113.28,7.62 | U3.15 113.53,7.87 v113.28,7.62 | U3.16 114.03,7.74 113.92,7.62 v113.28,7.62 | C5.2 119.08,8.85 | 119.08,8.85 119.76,8.75 C8.2 | R19.2 v119.25,7.37 119.08,8.85 | R15.2 v113.28,7.62 | v19.94,30.99 19.94,29.69 U11.10 | 96.32,7.67 96.27,8.13 | v55.12,88.71 D18:C5.1 54.98,90.42 53.59,90.42 D18:D41.1 | 49.33,100.64 49.28,100.58 | D16:C5.1 v54.61,100.01 | D0:C5.1 53.21,207.52 | 53.21,207.52 53.21,207.07 v53.34,206.95 | D0:D41.1 53.14,207.45 53.21,207.52 | D0:D31.1 49.34,209.11 49.28,209.04 | D2:D41.1 54.1,195.76 v54.86,196.02 | D4:D31.1 50.55,181.36 50.04,181.86 49.34,181.86 v49.28,181.8 | 53.96,181.86 53.34,181.86 53.09,181.61 D4:D41.1 | D3:D41.1 v100.84,193.74 | D3:D31.1 96.4,194.38 v96.27,194.25 | D5:D31.1 96.39,179.14 v96.27,179.26 | D5:D41.1 100.91,177.99 D5:C5.1 | D7:D31.1 v96.27,167.83 | D9:D31.1 97.54,155.19 v96.27,155.13 | D9:D41.1 100.33,154.43 D9:C5.1 | D11:D31.1 v96.27,142.43 | D11:D41.1 v101.35,140.91 | D12:D41.1 v101.35,133.03 | D12:D31.1 v96.27,132.27 | D14:D41.1 v100.84,116.01 | D14:D31.1 v96.27,117.03 | D17:D41.1 89.28,97.34 90.29,97.35 v90.55,97.35 | D17:D31.1 86.61,98.87 v85.47,98.87 | D10:D41.1 56.71,141.66 56.64,141.73
  Top 0.254: D10:D31.1 52.9,143.58 52.32,143 51.88,143 v51.82,143.06 | D13:D41.1 54.1,130.05 D13:C5.1 | D13:D31.1 50.04,131.06 v49.28,131 | D15:D31.1 v49.28,118.3 | D16:D31.1 50.16,101.73 v49.28,101.79 | D18:D31.1 50.16,90.68 v49.28,90.61 | D20:D41.1 54.36,74.68 55.12,74.68 | D20:D31.1 50.67,75 v50.55,75.12 | D31:D41.1 100.01,8.82 100.33,9.14 100.98,9.14 | 100.98,9.14 D31:C5.1 | D31:D31.1 97.61,10.48 97.28,10.16 97.28,9.65 96.77,9.14 96.33,9.14 v96.27,9.08 | 100.98,9.14 100.98,8.43 v101.35,8.06 | D22:C5.1 56.78,63.83 v56.64,63.69 56.13,63.18 D22:D41.1 | D22:D31.1 50.87,64.33 50.29,63.75 49.34,63.75 v49.28,63.69 | D28:D31.1 51.5,24.2 51.05,23.75 49.97,23.75 v49.91,23.69 | v56.01,22.48 55.12,23.37 D28:C5.1 54.88,24 54.23,24 54.1,23.37 D28:D41.1 | D26:D31.1 50.87,37.41 50.55,37.08 49.34,37.08 v49.28,37.02 | D26:C5.1 55.63,35.24 v55.37,34.99 55.31,35.05 54.1,35.05 53.09,36.07 D26:D41.1
  Top 0.305: R5.1 v12.32,186.69 C1.2 | U1.10 20.83,191.26 v21.21,191.77 | R11.1 54.86,186.69 v54.48,187.83 55.5,188.59 C2.2 | U2.10 v65.91,190.63 | R52.1 v121.54,130.18 | U14.7 123.7,124.97 | R54.1 v129.16,126.36 | U4.2 C6.2 v112.01,81.28 | U17.2 v125.09,71.12 123.46,71.12 R57.2 | C25.2 v130.3,68.58 C29.2 | v57.4,150.5 56.77,149.86 16.76,149.86 v15.49,151.13 | R29.1 11.67,77.45 v12.32,78.11 12.57,78.36 C11.2 | v55.75,73.41 56.39,74.04 C12.2 56.75,74.68 | R36.1 55.86,72.76 v55.75,73.41 | U10.10 63.88,76.71 v63.75,76.83 | v11.68,30.99 12.3,30.37 C13.2 12.32,28.84 R41.1 | C14.2 v56.01,22.48 55.99,22.46 R44.1 | U12.10 65.15,25.27 v65.02,25.4 | U6.10 20.7,140.46 v21.21,140.97 | v21.21,79.38 21.21,78.59 U9.10 | C10.2 v57.91,141.73 | R25.1 v57.91,141.73 | U7.10 v66.93,142.88 | v122.05,78.61 122.17,77.47 C19.2 | R1.1 108.97,117.35 107.95,117.35 106.43,115.82 | R22.1 C9.2 15.64,141.62 v15.75,141.73 | D5:C5.1 100.85,177.93 100.85,176.58 v100.97,176.47 | 96.03,177.29 D5:R48.1 | D3:C5.1 v100.84,193.74 | D12:C5.1 v101.35,133.03 | D6:C5.1 54.1,168.97 v54.23,167.32 53.46,167.32 D6:D41.1 | D2:C5.1 55.29,196.96 v54.86,196.02 | 53.96,181.86 D4:C5.1 54.1,180.53 v54.67,180.09 | 49.33,180.39 49.28,180.34 | v55.75,73.41 55.12,74.04 55.12,74.68 D20:C5.1 55.01,75.44 | 50.6,74.22 50.55,74.17 | 54.01,156.92 D8:C5.1 v53.97,155.13 53.08,155.13 D8:D41.1 | 56.64,141.73 v57.91,141.73 | D10:C5.1 v57.91,141.73 | 96.18,166.17 D7:R48.1 | D7:C5.1 v101.6,165.93 101.54,165.86 100.97,165.86 100.65,166.17 D7:D41.1 | D17:C5.1 90.68,98.49 v90.55,97.35 | 48.99,129.08 D13:R48.1 | D13:C5.1 v54.74,128.97 | 49.33,116.89 49.28,116.84 | D15:C5.1 54.48,117.79 54.44,117.42 v54.48,116.52 D15:D41.1
  Top 0.305: 101.76,206.2 D1:C5.1 101.85,204.91 v101.73,204.79 101.66,204.72 100.84,204.72 D1:D41.1 | 95.98,204.27 D1:R48.1 | 96.12,153.42 D9:R48.1 | D9:C5.1 v101.6,152.72 | 96.3,140.89 D11:R48.1 | D11:C5.1 v101.35,140.91 | 100.75,117.3 D14:C5.1 v100.84,116.01 | 96.18,115.37 D14:R48.1 | D2:D31.1 49.33,196.41 49.28,196.47 | D1:D31.1 97.61,206.57 97.28,206.25 96.33,206.25 v96.27,206.19 | D6:D31.1 50.67,169.1 v49.28,169.1 | D8:D31.1 50.1,156.46 50.04,156.46 49.97,156.4 v49.28,156.4 | D24:D41.1 53.16,47.43 D24:C5.1 53.34,47.61 v53.34,45.91 | D24:D31.1 49.33,49.09 49.28,49.15 | D30:D31.1 50.17,12.52 v49.91,12.26 | D30:D41.1 53.72,10.41 55.43,10.41 v55.5,10.35 55.63,10.48 D30:C5.1 | D19:D41.1 89.67,86.8 v90.55,85.92 91,86.36 91.19,86.36 91.55,86.73 D19:C5.1 | D19:D31.1 87.06,88.21 86.23,87.38 85.54,87.38 v85.47,87.44 | D21:D31.1 93.73,73.41 92.96,72.64 92.52,72.64 v92.46,72.58 | D21:D41.1 95.76,70.8 v97.28,71.31 97.59,71.61 D21:C5.1 | v101.85,58.61 D23:C5.1 101.67,60.13 D23:D41.1 | D23:D31.1 96.4,61.28 v96.27,61.15 | D25:D31.1 97.79,46.99 97.16,46.35 96.33,46.35 v96.27,46.42 | D25:C5.1 102.18,45.91 102.18,44.57 v101.35,44.39 100.84,44.89 D25:D41.1 | D27:C5.1 v103.38,34.48 102.1,34.22 D27:D41.1 | D27:D31.1 99.82,35.69 99.06,34.92 96.33,34.92 v96.27,34.99 | D29:D41.1 v100.97,18.35 101.85,19.24 D29:C5.1 | D29:D31.1 97.61,21.15 97.28,20.83 96.33,20.83 v96.27,20.77 | U14.6 128.63,124.82 128.78,124.97 | C17.+ 115.06,120.42 115.06,120.4 | D16:D41.1 v54.6,100.01 v54.61,100.01
  Top 0.406: D0:R46.1 v24.83,208.15 | D0:C46.2 30.76,209.11 | 30.76,209.11 D0:C36.2 | D0:C42.1 34.67,209.11 | 34.67,209.11 D0:C32.1 | 34.67,209.11 v32.45,209.11 30.76,209.11 | D1:R46.1 v71.82,205.87 | D1:C46.2 77.75,206.82 | 77.75,206.82 D1:C36.2 | D1:C42.1 81.66,206.82 | 81.66,206.82 D1:C32.1 | 81.66,206.82 v79.44,206.82 77.75,206.82 | D2:R46.1 v24.83,196.72 | D2:C46.2 30.76,197.68 | 30.76,197.68 D2:C36.2 | D2:C42.1 34.67,197.68 | 34.67,197.68 D2:C32.1 | 34.67,197.68 v32.45,197.68 30.76,197.68 | D3:R46.1 v71.82,193.93 | D3:C46.2 77.75,194.88 | 77.75,194.88 D3:C36.2 | D3:C42.1 81.66,194.88 | 81.66,194.88 D3:C32.1 | 81.66,194.88 v79.44,194.88 77.75,194.88 | D4:R46.1 v24.83,181.48 | D4:C46.2 30.76,182.44 | 30.76,182.44 D4:C36.2 | D4:C42.1 34.67,182.44 | 34.67,182.44 D4:C32.1 | 34.67,182.44 v32.45,182.44 30.76,182.44 | D5:R46.1 v71.82,178.94 | D5:C46.2 77.75,179.9 | 77.75,179.9 D5:C36.2 | D5:C42.1 81.66,179.9 | 81.66,179.9 D5:C32.1 | 81.66,179.9 v79.44,179.9 77.75,179.9 | D6:R46.1 v24.83,168.78 | D6:C46.2 30.76,169.74 | 30.76,169.74 D6:C36.2 | D6:C42.1 34.67,169.74 | 34.67,169.74 D6:C32.1 | 34.67,169.74 v32.45,169.74 30.76,169.74 | D7:R46.1 v71.82,167.51 | D7:C46.2 77.75,168.47 | 77.75,168.47 D7:C36.2 | D7:C42.1 81.66,168.47 | 81.66,168.47 D7:C32.1 | 81.66,168.47 v79.44,168.47 77.75,168.47 | D8:R46.1 v24.83,156.08 | D8:C46.2 30.76,157.04 | 30.76,157.04 D8:C36.2 | D8:C42.1 34.67,157.04 | 34.67,157.04 D8:C32.1 | 34.67,157.04 v32.45,157.04 30.76,157.04 | D9:R46.1 v71.82,154.81 | D9:C46.2 77.75,155.77 | 77.75,155.77 D9:C36.2 | D9:C42.1 81.66,155.77 | 81.66,155.77 D9:C32.1 | 81.66,155.77 v79.44,155.77 77.75,155.77 | D10:R46.1 v27.37,142.75 | D10:C46.2 33.3,143.7 | 33.3,143.7 D10:C36.2
  Top 0.406: D10:C42.1 37.21,143.7 | 37.21,143.7 D10:C32.1 | 37.21,143.7 v34.99,143.7 33.3,143.7 | D11:R46.1 v71.82,142.11 | D11:C46.2 77.75,143.06 | 77.75,143.06 D11:C36.2 | D11:C42.1 81.66,143.06 | 81.66,143.06 D11:C32.1 | 81.66,143.06 v79.44,143.06 77.75,143.06 | D13:R46.1 v24.83,130.68 | D13:C46.2 30.76,131.64 | 30.76,131.64 D13:C36.2 | D13:C42.1 34.67,131.64 | 34.67,131.64 D13:C32.1 | 34.67,131.64 v32.45,131.64 30.76,131.64 | D12:R46.1 v71.82,131.95 | D12:C46.2 77.75,132.91 | 77.75,132.91 D12:C36.2 | D12:C42.1 81.66,132.91 | 81.66,132.91 D12:C32.1 | 81.66,132.91 v79.44,132.91 77.75,132.91 | D15:R46.1 v24.83,117.98 | D15:C46.2 30.76,118.94 | 30.76,118.94 D15:C36.2 | D15:C42.1 34.67,118.94 | 34.67,118.94 D15:C32.1 | 34.67,118.94 v32.45,118.94 30.76,118.94 | D14:R46.1 v71.82,116.71 | D14:C46.2 77.75,117.67 | 77.75,117.67 D14:C36.2 | D14:C42.1 81.66,117.67 | 81.66,117.67 D14:C32.1 | 81.66,117.67 v79.44,117.67 77.75,117.67 | D16:R46.1 v24.83,101.47 | D16:C46.2 30.76,102.42 | 30.76,102.42 D16:C36.2 | D16:C42.1 34.67,102.42 | 34.67,102.42 D16:C32.1 | 34.67,102.42 v32.45,102.42 30.76,102.42 | D17:R46.1 v61.02,98.55 | D17:C46.2 66.95,99.5 | 66.95,99.5 D17:C36.2 | D17:C42.1 70.87,99.5 | 70.87,99.5 D17:C32.1 | 70.87,99.5 v68.64,99.5 66.95,99.5 | D18:R46.1 v24.83,90.3 | D18:C46.2 30.76,91.25 | 30.76,91.25 D18:C36.2 | D18:C42.1 34.67,91.25 | 34.67,91.25 D18:C32.1 | 34.67,91.25 v32.45,91.25 30.76,91.25 | D19:R46.1 v61.02,87.12 | D19:C46.2 66.95,88.08 | 66.95,88.08 D19:C36.2 | D19:C42.1 70.87,88.08 | 70.87,88.08 D19:C32.1 | 70.87,88.08 v68.64,88.08 66.95,88.08 | D20:R46.1 v26.1,74.8 | D20:C46.2 32.03,75.75 | 32.03,75.75 D20:C36.2 | D20:C42.1 35.94,75.75 | 35.94,75.75 D20:C32.1 | 35.94,75.75 v33.72,75.75 32.03,75.75
  Top 0.406: D21:R46.1 v68.01,72.26 | D21:C46.2 73.94,73.22 | 73.94,73.22 D21:C36.2 | D21:C42.1 77.85,73.22 | 77.85,73.22 D21:C32.1 | 77.85,73.22 v75.63,73.22 73.94,73.22 | D22:R46.1 v24.83,63.37 | D22:C46.2 30.76,64.33 | 30.76,64.33 D22:C36.2 | D22:C42.1 34.67,64.33 | 34.67,64.33 D22:C32.1 | 34.67,64.33 v32.45,64.33 30.76,64.33 | D23:R46.1 v71.82,60.83 | D23:C46.2 77.75,61.78 | 77.75,61.78 D23:C36.2 | D23:C42.1 81.66,61.78 | 81.66,61.78 D23:C32.1 | 81.66,61.78 v79.44,61.78 77.75,61.78 | D24:R46.1 v24.83,48.13 | D24:C46.2 30.76,49.09 | 30.76,49.09 D24:C36.2 | D24:C42.1 34.67,49.09 | 34.67,49.09 D24:C32.1 | 34.67,49.09 v32.45,49.09 30.76,49.09 | D25:R46.1 v71.82,46.1 | D25:C46.2 77.75,47.05 | 77.75,47.05 D25:C36.2 | D25:C42.1 81.66,47.05 | 81.66,47.05 D25:C32.1 | 81.66,47.05 v79.44,47.05 77.75,47.05 | D26:R46.1 v24.83,36.7 | D26:C46.2 30.76,37.66 | 30.76,37.66 D26:C36.2 | D26:C42.1 34.67,37.66 | 34.67,37.66 D26:C32.1 | 34.67,37.66 v32.45,37.66 30.76,37.66 | D27:R46.1 v71.82,34.67 | D27:C46.2 77.75,35.62 | 77.75,35.62 D27:C36.2 | D27:C42.1 81.66,35.62 | 81.66,35.62 D27:C32.1 | 81.66,35.62 v79.44,35.62 77.75,35.62 | D28:R46.1 v25.46,23.37 | D28:C46.2 31.39,24.32 | 31.39,24.32 D28:C36.2 | D28:C42.1 35.31,24.32 | 35.31,24.32 D28:C32.1 | 35.31,24.32 v33.08,24.32 31.39,24.32 | D29:R46.1 v71.82,20.45 | D29:C46.2 77.75,21.4 | 77.75,21.4 D29:C36.2 | D29:C42.1 81.66,21.4 | 81.66,21.4 D29:C32.1 | 81.66,21.4 v79.44,21.4 77.75,21.4 | D30:R46.1 v25.46,11.94 | D30:C46.2 31.39,12.89 | 31.39,12.89 D30:C36.2 | D30:C42.1 35.31,12.89 | 35.31,12.89 D30:C32.1 | 35.31,12.89 v33.08,12.89 31.39,12.89 | D31:R46.1 v71.82,8.76 | D31:C46.2 77.75,9.72 | 77.75,9.72 D31:C36.2 | D31:C42.1 81.66,9.72 | 81.66,9.72 D31:C32.1
  Top 0.406: 81.66,9.72 v79.44,9.72 77.75,9.72 | C37.2 117.09,15.88 117.73,16.51 T2.TP | U19.2 121.03,192.41 121.54,191.9 v121.54,191.13 v121.52,191.12 C26.2 | C24.2 v112.65,191.77 | R59.2 v125.98,192.41 | C27.2 113.9,7 v113.28,7.62 | C23.2 121.54,89.53 v120.9,90.17 | C22.2 v122.17,206.38 | C28.1 129.46,115.49 v129.39,114.55 | OK1.2 v128.27,27.43
  Top 0.61: 123.7,124.97 123.44,125.73 v122.81,125.73 | C15.1 v116.71,120.27 116.84,120.4 115.06,120.4 | 128.78,124.97 128.78,125.98 v129.16,126.36
  Top 0.813: C16.- 112.52,93.98 | 112.52,93.98 v111.38,93.98 | 103.38,106.68 103.15,106.45 C18.- 101.35,106.58 D41.A | D43.C 107.44,120.3 v107.44,120.52 | 113.03,91.44 D42.A 112.52,91.44 112.52,93.98 | D44.A 135.38,102.11 135.38,104.78 | D45.C 141.99,118.36 v141.99,118.49
  Top 1.016: 132.97,122.56 C21.+ v134.87,122.05 | C4.- 135.38,104.78 v136.14,104.78
  Route2 0.61: v129.16,126.36 127.89,125.09 124.08,125.09 123.44,125.73 v122.81,125.73
  BOTTOM 0.254: v128.27,27.43 127.25,28.96
  BOTTOM 0.406: v24.83,208.15 25.15,208.79 | v71.82,205.87 72.14,206.5 | v24.83,196.72 25.15,197.36 | v71.82,193.93 72.14,194.56 | v24.83,181.48 25.15,182.12 | v71.82,178.94 72.14,179.58 | v24.83,168.78 25.15,169.42 | v71.82,167.51 72.14,168.15 | v24.83,156.08 25.15,156.72 | v71.82,154.81 72.14,155.45 | v27.37,142.75 27.69,143.38 | v71.82,142.11 72.14,142.75 | v24.83,130.68 25.15,131.32 | v71.82,131.95 72.14,132.59 | v24.83,117.98 25.15,118.62 | v71.82,116.71 72.14,117.35 | v24.83,101.47 25.15,102.11 | v61.02,98.55 61.34,99.19 | v24.83,90.3 25.15,90.93 | v61.02,87.12 61.34,87.76 | v26.1,74.8 26.42,75.44 | v68.01,72.26 68.33,72.9 | v24.83,63.37 25.15,64.01 | v71.82,60.83 72.14,61.47 | v24.83,48.13 25.15,48.77 | v71.82,46.1 72.14,46.74 | v24.83,36.7 25.15,37.34 | v71.82,34.67 72.14,35.31 | v25.46,23.37 25.78,24 | v71.82,20.45 72.14,21.08 | v25.46,11.94 25.78,12.57 | v71.82,8.76 72.14,9.4
  other vias: 106.3,108.58 105.66,102.23 116.84,105.03 124.71,109.22 124.71,114.94 122.81,114.94 115.82,114.94 104.39,114.94 104.39,104.14 106.3,104.78 120.9,98.42 122.81,98.42 122.81,92.71 120.9,92.71 122.81,90.17 115.19,111.76 125.35,97.79 124.71,94.61 125.98,90.81 129.16,90.81 131.06,90.17 133.6,98.42 131.06,99.06 113.28,10.16 115.19,108.58 110.34,109.78 114.81,105.03
  pour BOTTOM: 24.51,213.23 24.51,204.34 49.91,204.34 49.91,213.23
  pour BOTTOM: 71.5,210.95 71.5,202.06 96.9,202.06 96.9,210.95
  pour BOTTOM: 24.51,201.8 24.51,192.91 49.91,192.91 49.91,201.8
  pour BOTTOM: 71.5,199.01 71.5,190.12 96.9,190.12 96.9,199.01
  pour BOTTOM: 24.51,186.56 24.51,177.67 49.91,177.67 49.91,186.56
  pour BOTTOM: 71.5,184.02 71.5,175.13 96.9,175.13 96.9,184.02
  pour BOTTOM: 24.51,173.86 24.51,164.97 49.91,164.97 49.91,173.86
  pour BOTTOM: 71.5,172.59 71.5,163.7 96.9,163.7 96.9,172.59
  pour BOTTOM: 24.51,161.16 24.51,152.27 49.91,152.27 49.91,161.16
  pour BOTTOM: 71.5,159.89 71.5,151 96.9,151 96.9,159.89
  pour BOTTOM: 27.05,147.83 27.05,138.94 52.45,138.94 52.45,147.83
  pour BOTTOM: 71.5,147.19 71.5,138.3 96.9,138.3 96.9,147.19
  pour BOTTOM: 24.51,135.76 24.51,126.87 49.91,126.87 49.91,135.76
  pour BOTTOM: 71.5,137.03 71.5,128.14 96.9,128.14 96.9,137.03
  pour BOTTOM: 24.51,123.06 24.51,114.17 49.91,114.17 49.91,123.06
  pour BOTTOM: 71.5,121.79 71.5,112.9 96.9,112.9 96.9,121.79
  pour BOTTOM: 24.51,106.55 24.51,97.66 49.91,97.66 49.91,106.55
  pour BOTTOM: 60.71,103.63 60.71,94.74 86.11,94.74 86.11,103.63
  pour BOTTOM: 24.51,95.38 24.51,86.49 49.91,86.49 49.91,95.38
  pour BOTTOM: 60.71,92.2 60.71,83.31 86.11,83.31 86.11,92.2
  pour BOTTOM: 25.78,79.88 25.78,70.99 51.18,70.99 51.18,79.88
  pour BOTTOM: 67.69,77.34 67.69,68.45 93.09,68.45 93.09,77.34
  pour BOTTOM: 24.51,68.45 24.51,59.56 49.91,59.56 49.91,68.45
  pour BOTTOM: 71.5,65.91 71.5,57.02 96.9,57.02 96.9,65.91
  pour BOTTOM: 24.51,53.21 24.51,44.32 49.91,44.32 49.91,53.21
  pour BOTTOM: 71.5,51.18 71.5,42.29 96.9,42.29 96.9,51.18
  pour BOTTOM: 24.51,41.78 24.51,32.89 49.91,32.89 49.91,41.78
  pour BOTTOM: 71.5,39.75 71.5,30.86 96.9,30.86 96.9,39.75
  pour BOTTOM: 25.15,28.45 25.15,19.56 50.55,19.56 50.55,28.45
  pour BOTTOM: 71.5,25.53 71.5,16.64 96.9,16.64 96.9,25.53
  pour BOTTOM: 25.15,17.02 25.15,8.13 50.55,8.13 50.55,17.02
  pour BOTTOM: 71.5,13.84 71.5,4.95 96.9,4.95 96.9,13.84
  pour Top (rank 3, no thermals): 110.11,116.2 113.92,116.2 113.77,100.56 109.93,100.63
  pour Top: 118.36,116.2 125.98,116.2 125.98,102.23 118.36,102.23
  pour Top (rank 3, no thermals): 103.12,116.2 110.11,116.2 110.36,100.58 103.12,100.58
  pour Top (no thermals): 119.63,99.69 127.25,99.69 127.25,88.9 119.63,88.9
  pour Top: 127.25,99.69 135.51,99.69 135.51,88.9 127.25,88.9
  pour Top (rank 3, no thermals): 113.92,116.2 118.36,116.2 118.36,102.23 113.92,102.23
  pour BOTTOM (no thermals): 113.92,116.2 118.36,116.2 118.36,102.23 113.92,102.23
  pour BOTTOM (no thermals): 119.63,99.69 127.25,99.69 127.25,88.9 119.63,88.9
  pour BOTTOM (rank 3): 2.79,217.81 145.67,217.81 146.94,216.53 146.94,1.91 2.79,1.91
  pour BOTTOM (no thermals): 123.42,100.71 102.97,100.71 102.97,116.23 126.03,116.23 126.03,116.03 126.11,116.03 126.11,104.57
  pour Top (rank 2): 107.44,109.22 111,109.22 111,107.19 107.44,107.19
GPIO2
  Top 0.305: GPIO2.TP X3.C26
